// ================================================================================
// Automatisch generiert vom S5/S7 Konverter,  Version K2.1.9.0-REL   29-03-2001 18:57
// ================================================================================
//
//                       Hinweise:
//                       ---------
//
// BAUSTEINE:       In S7 gibt es folgende Bausteintypen:
//OB: analog zu S5;
//FB: FunctionBlock (z.B. Regler), wird mit unterschiedlichen Instanz-DB's aufgerufen;
//FC: FunctionCall, vergleichbar mit FB von S5.
//Die Bausteintypen PB, FX, DX und SB entfallen.
//
//OB'S:   OB's können in S7 nicht vom Anwenderprogramm aus aufgerufen werden.
//        Sonderfunktions-OB's werden, analog zu Spezialbefehlen wie z.B. E  DB,
//             durch neue Befehle oder durch SFC's ersetzt.
//
// ADRESSIERUNG: In S7 werden alle Speicherbereiche (E, A, M, D, usw.) einheitlich
//             byteweise adressiert. D.h. aus  L  DW 2 in S5 wird  L  DBW 4 in S7.
//
// AKKU-ANZAHL: S7-CPU's besitzen wie S5-CPU's 2 oder 4 Akkus.
//              Wird ein S5-Programm von einer S5-CPU mit 2 Akkus (115U) für eine S7-CPU
//              mit 4 Akkus konvertiert, so muß vor jeder arithmetischen Operation
//             (+,-,*,/) der ENT-Befehl eingefügt werden, falls danach der Inhalt von Akku2
//              weiterverwendet werden soll.
//
// AKKU-BREITE: Die Akkus aller S7-CPU's sind 32-Bit breit.
//              Bei Festpunktrechenbefehlen in S7
//              - bleibt bei Über- / Unterlauf das Highwort von Akku1 unverändert
//                (135U : Vorzeichen);
//              - wird keine implizite Wandlung nach 32-Bit Format durchgeführt (155U).
//
// OS-BIT:      Bei den folgenden Operationen bleibt in S7 das OS-Bit
//             (Überlauf speichernd) unverändert (wurde in S5 zurückgesetzt):
//             T,  >F, <F, ><F, !=F, >=F, <=F,  >D, <D, ><D, !=D, >=D, <=D,
//             >G, <G, ><G, !=G, >=G, <=G,
//             SLW, SRW, SLD, SVW, SVD, RLD, RRD
//
// OV-BIT:      Die folgenden Wandlungsoperationen belassen den Akku1
//              bei Überlauf unverändert (in S5: Betrag der Festpunktzahl).
//              Ein Überlauf wird im OS- und OV-Bit (S5: nur OS) angezeigt.
//              DUF, DUD, GFD
//
// LIR, TIR:    In S7 gibt es keine absolut adressierenden Befehle. Sie sind
//              teilweise durch neue Befehle (z.B. Zugriff auf Datenworte größer als 255),
//              teilweise  durch Systemfunctions (SFC) zu ersetzen. Gleiches gilt für
//              Datenbausteinanfangs-,Datenbausteinlängen- und Basisregister.
//
// DATENBEREICHE BS,BT,BA,BB,Q:
//              Bei Verwendung dieser Datenbereiche muß manuell eingegriffen werden.
//              Mögliche Lösungen :
//                 - Vergrößerten Merkerbereich verwenden
//                 - Längere Datenbausteine definieren
//                 - S7 System Functions einsetzen
//
// STOPPBEFEHLE: In S7 gibt es nur noch eine Stoppanweisung, mittels SFC-Aufruf
//               ausführbar. Er entspricht dem STS-Befehl von S5.
//
// Bei weiteren Fragen siehe Handbuch oder Online-Hilfe.

FUNCTION FC 0 : VOID
  BEGIN
  NETWORK
  TITLE = SIEBEN-SEGMENT-ANZEIGE
       NOP 0;
  NETWORK
  TITLE = ZAHLENAUSWERTUNG ZAHL 0
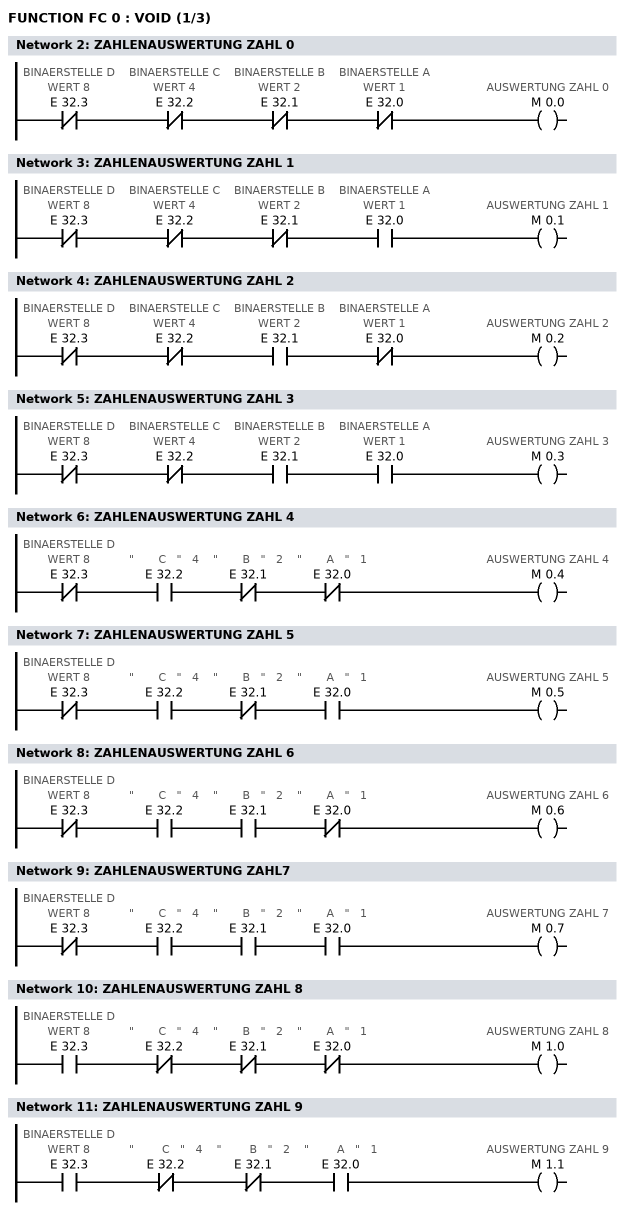
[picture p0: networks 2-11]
       UN  E 32.3;               // BINAERSTELLE D  WERT 8
       UN  E 32.2;               // BINAERSTELLE C  WERT 4
       UN  E 32.1;               // BINAERSTELLE B  WERT 2
       UN  E 32.0;               // BINAERSTELLE A  WERT 1
       =   M 0.0;                // AUSWERTUNG ZAHL 0
  NETWORK
  TITLE = ZAHLENAUSWERTUNG ZAHL 1
       UN  E 32.3;               // BINAERSTELLE D  WERT 8
       UN  E 32.2;               // BINAERSTELLE C  WERT 4
       UN  E 32.1;              // BINAERSTELLE B  WERT 2
       U   E 32.0;              // BINAERSTELLE A  WERT 1
       =   M 0.1;               // AUSWERTUNG ZAHL 1
  NETWORK
  TITLE = ZAHLENAUSWERTUNG ZAHL 2
       UN  E 32.3;              // BINAERSTELLE D  WERT 8
       UN  E 32.2;              // BINAERSTELLE C  WERT 4
       U   E 32.1;              // BINAERSTELLE B  WERT 2
       UN  E 32.0;              // BINAERSTELLE A  WERT 1
       =   M 0.2;               // AUSWERTUNG ZAHL 2
  NETWORK
  TITLE = ZAHLENAUSWERTUNG ZAHL 3
       UN  E 32.3;              // BINAERSTELLE D  WERT 8
       UN  E 32.2;              // BINAERSTELLE C  WERT 4
       U   E 32.1;              // BINAERSTELLE B  WERT 2
       U   E 32.0;              // BINAERSTELLE A  WERT 1
       =   M 0.3;               // AUSWERTUNG ZAHL 3
  NETWORK
  TITLE = ZAHLENAUSWERTUNG ZAHL 4
       UN  E 32.3;              // BINAERSTELLE D  WERT 8
       U   E 32.2;              //      "       C   "   4
       UN  E 32.1;              //      "       B   "   2
       UN  E 32.0;              //      "       A   "   1
       =   M 0.4;               // AUSWERTUNG ZAHL 4
  NETWORK
  TITLE = ZAHLENAUSWERTUNG ZAHL 5
       UN  E 32.3;              // BINAERSTELLE D  WERT 8
       U   E 32.2;              //      "       C   "   4
       UN  E 32.1;              //      "       B   "   2
       U   E 32.0;              //      "       A   "   1
       =   M 0.5;               // AUSWERTUNG ZAHL 5
  NETWORK
  TITLE = ZAHLENAUSWERTUNG ZAHL 6
       UN  E 32.3;              // BINAERSTELLE D  WERT 8
       U   E 32.2;              //      "       C   "   4
       U   E 32.1;              //      "       B   "   2
       UN  E 32.0;              //      "       A   "   1
       =   M 0.6;               // AUSWERTUNG ZAHL 6
  NETWORK
  TITLE = ZAHLENAUSWERTUNG ZAHL7
       UN  E 32.3;              // BINAERSTELLE D  WERT 8
       U   E 32.2;              //      "       C   "   4
       U   E 32.1;              //      "       B   "   2
       U   E 32.0;              //      "       A   "   1
       =   M 0.7;               // AUSWERTUNG ZAHL 7
  NETWORK
  TITLE = ZAHLENAUSWERTUNG ZAHL 8
       U   E 32.3;              // BINAERSTELLE D  WERT 8
       UN  E 32.2;              //      "       C   "   4
       UN  E 32.1;              //      "       B   "   2
       UN  E 32.0;              //      "       A   "   1
       =   M 1.0;               // AUSWERTUNG ZAHL 8
  NETWORK
  TITLE = ZAHLENAUSWERTUNG ZAHL 9
       U   E 32.3;              // BINAERSTELLE D  WERT 8
       UN  E 32.2;              //     "        C   "   4
       UN  E 32.1;              //     "        B   "   2
       U   E 32.0;              //     "        A   "   1
       =   M 1.1;               // AUSWERTUNG ZAHL 9
  NETWORK
  TITLE = SEGMENTANSTEUERUNG
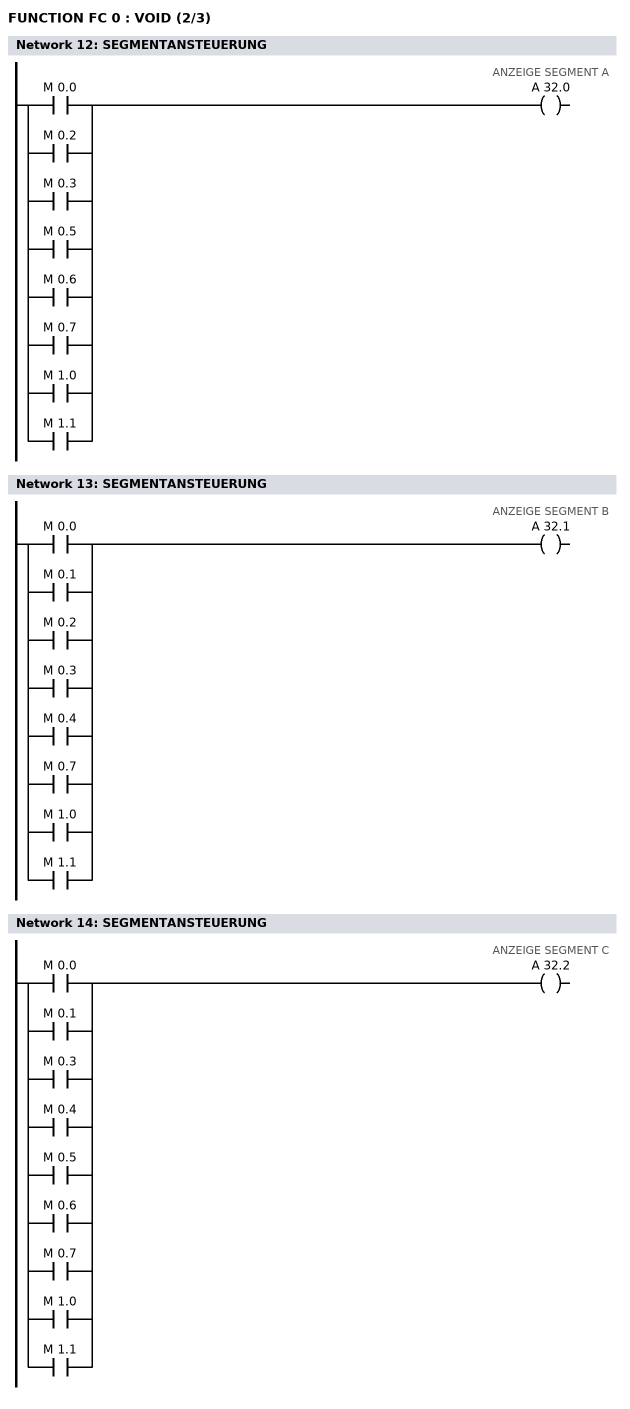
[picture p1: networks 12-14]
       O   M 0.0;
       O   M 0.2;
       O   M 0.3;
       O   M 0.5;
       O   M 0.6;
       O   M 0.7;
       O   M 1.0;
       O   M 1.1;
       =   A 32.0;              // ANZEIGE SEGMENT A
  NETWORK
  TITLE = SEGMENTANSTEUERUNG
       O   M 0.0;
       O   M 0.1;
       O   M 0.2;
       O   M 0.3;
       O   M 0.4;
       O   M 0.7;
       O   M 1.0;
       O   M 1.1;
       =   A 32.1;              // ANZEIGE SEGMENT B
  NETWORK
  TITLE = SEGMENTANSTEUERUNG
       O   M 0.0;
       O   M 0.1;
       O   M 0.3;
       O   M 0.4;
       O   M 0.5;
       O   M 0.6;
       O   M 0.7;
       O   M 1.0;
       O   M 1.1;
       =   A 32.2;              // ANZEIGE SEGMENT C
  NETWORK
  TITLE = SEGMENTANSTEUERUNG
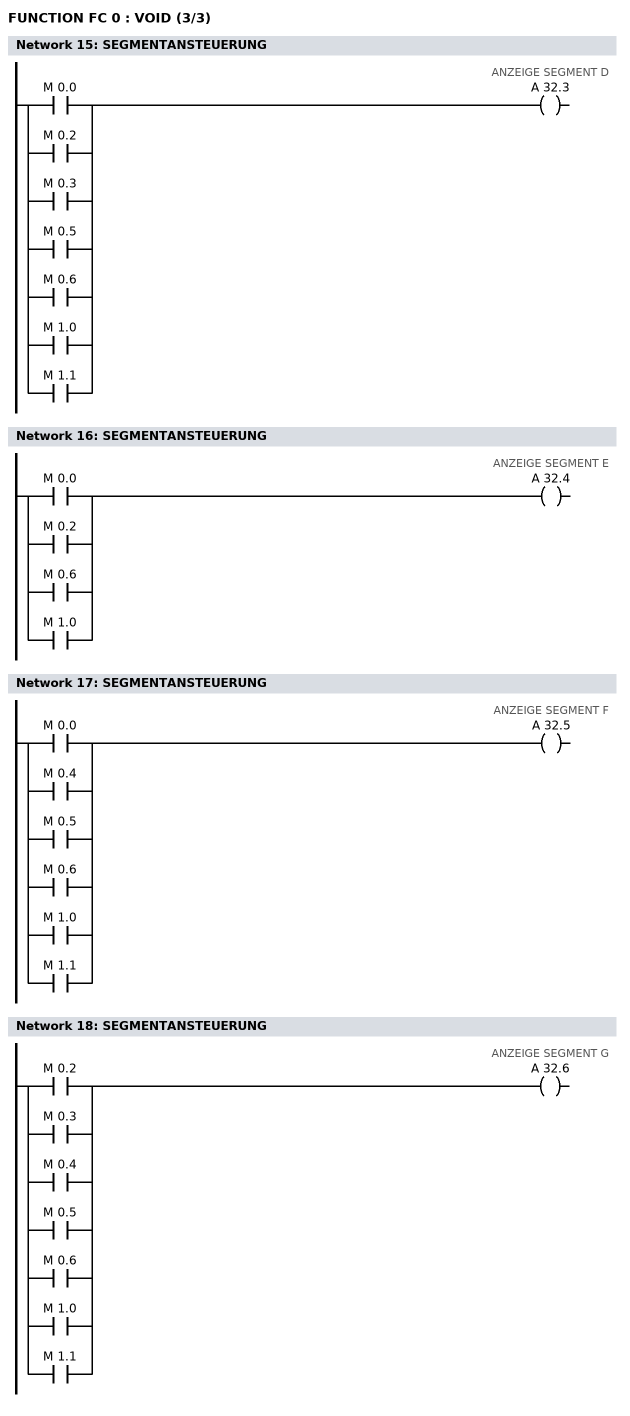
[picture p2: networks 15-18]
       O   M 0.0;
       O   M 0.2;
       O   M 0.3;
       O   M 0.5;
       O   M 0.6;
       O   M 1.0;
       O   M 1.1;
       =   A 32.3;             // ANZEIGE SEGMENT D
  NETWORK
  TITLE = SEGMENTANSTEUERUNG
       O   M 0.0;
       O   M 0.2;
       O   M 0.6;
       O   M 1.0;
       =   A 32.4;             // ANZEIGE SEGMENT E
  NETWORK
  TITLE = SEGMENTANSTEUERUNG
       O   M 0.0;
       O   M 0.4;
       O   M 0.5;
       O   M 0.6;
       O   M 1.0;
       O   M 1.1;
       =   A 32.5;             // ANZEIGE SEGMENT F
  NETWORK
  TITLE = SEGMENTANSTEUERUNG
       O   M 0.2;
       O   M 0.3;
       O   M 0.4;
       O   M 0.5;
       O   M 0.6;
       O   M 1.0;
       O   M 1.1;
       =   A 32.6;             // ANZEIGE SEGMENT G


END_FUNCTION
